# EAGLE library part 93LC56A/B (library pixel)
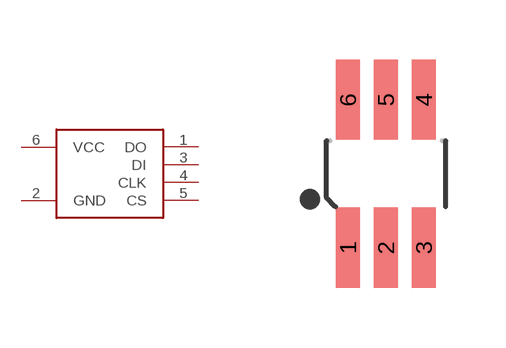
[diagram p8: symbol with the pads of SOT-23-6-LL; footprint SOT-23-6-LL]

Designator prefix -

## 93LC56A/B  [SOT-23-6-LL]
1  DO
2  GND
3  DI
4  CLK
5  CS
6  VCC

## Footprint SOT-23-6-LL (pad centres in mm)
smd 0.6 x 2: 1 -0.95,-1.85; 2 0,-1.85; 3 0.95,-1.85; 4 0.95,1.85; 5 0,1.85; 6 -0.95,1.85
